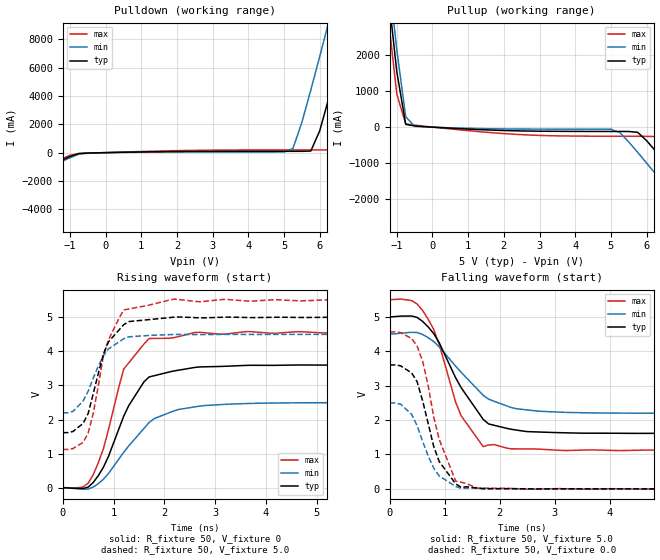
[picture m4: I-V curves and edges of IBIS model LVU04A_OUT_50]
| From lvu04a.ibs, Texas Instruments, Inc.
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|   Model LVU04A_OUT_50
[Model]   LVU04A_OUT_50
Model_type  Output
Polarity   Inverting
Vmeas = 2.50v
Cref = 15pf
| variable   typ   min   max
C_comp   6.50pf   4.88pf   8.13pf
[Temperature Range]   25   85   -40
[Voltage Range]   5.0   4.5   5.5
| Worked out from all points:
|   slope of the pulldown table from 0 to 0.75 V, typ, clamps not added: 19.9 ohm
|   slope of the pullup table from 0 to 0.75 V, typ, clamps not added: 17.9 ohm
|   rising waveform, R_fixture 50, V_fixture 0: 20-80 % time 664ps typ, 834ps min, 547ps max; typ from 0 V to 3.6 V
|   falling waveform, R_fixture 50, V_fixture 5.0: 20-80 % time 709ps typ, 805ps min, 553ps max; typ from 5 V to 1.61 V
|   rising waveform, R_fixture 50, V_fixture 5.0: 20-80 % time 405ps typ, 443ps min, 425ps max; typ from 1.61 V to 5 V
|   falling waveform, R_fixture 50, V_fixture 0.0: 20-80 % time 394ps typ, 395ps min, 422ps max; typ from 3.6 V to 0 V
[Pulldown]
|   Voltage   I(typ)   I(min)   I(max)
-5V       -5.137A    -5.221A    -5.049A
-750mV    -58.91mA   -107.9mA   -71.34mA
5V        93.29mA    48.15mA    192mA
5.25V     93.34mA    298.4mA    192.2mA
5.75V     115.9mA    4.416A     192.3mA
6V        1.543A     6.782A     192.5mA
6.25V     3.802A     9.188A     193.6mA
6.5V      6.175A     11.62A     931.3mA
6.75V     8.589A     14.06A     3.152A
7.25V     13.47A     18.96A     7.958A
7.5V      15.93A     21.43A     10.4A
10V       40.69A     46.19A     35.16A
[Pullup]
|   Voltage   I(typ)   I(min)   I(max)
-5V       40.69A     41.22A     40.13A
-1.25V    3.8A       4.415A     3.147A
-1V       1.538A     2.141A     913.8mA
-750mV    77.31mA    289.2mA    88.2mA
-500mV    33.52mA    21.54mA    56.26mA
5V        -119.7mA   -57.82mA   -252.2mA
5.75V     -143.8mA   -698.4mA   -252.6mA
6.25V     -660.6mA   -1.294A    -261mA
7.5V      -2.169A    -2.814A    -1.581A
8V        -2.781A    -3.427A    -2.192A
8.5V      -3.395A    -4.041A    -2.806A
10V       -5.243A    -5.888A    -4.654A
[Ramp]
| variable   typ   min   max
dV/dt_r  2.1615E+00/6.4572E-10  1.4987E+00/8.5844E-10  2.7383E+00/5.0255E-10
dV/dt_f  2.0525E+00/6.3930E-10  1.4118E+00/8.3550E-10  2.6399E+00/5.4668E-10
R_load = 50
[Rising Waveform]
R_fixture = 50
V_fixture = 0
|   Time   V(typ)   V(min)   V(max)
0s        0V         0V         0V
400ps     -27.85mV   -45.29mV   16mV
600ps     151.8mV    16.63mV    380.7mV
800ps     599mV      246.5mV    1.142V
1.2ns     2.099V     1.038V     3.482V
1.6ns     3.11V      1.741V     4.22V
1.8ns     3.287V     2.027V     4.381V
2.6ns     3.53V      2.372V     4.554V
4.8ns     3.601V     2.492V     4.57V
25ns      3.602V     2.498V     4.561V
[Falling Waveform]
R_fixture = 50
V_fixture = 5.0
V_fixture_min = 4.5
V_fixture_max = 5.5
|   Time   V(typ)   V(min)   V(max)
0s        5V         4.5V       5.5V
400ps     5.026V     4.552V     5.475V
600ps     4.869V     4.489V     5.184V
900ps     4.252V     4.132V     4.209V
1.2ns     3.228V     3.567V     2.518V
1.3ns     2.942V     3.389V     2.124V
1.7ns     2.021V     2.72V      1.229V
2.3ns     1.711V     2.331V     1.163V
3.7ns     1.619V     2.208V     1.133V
25ns      1.614V     2.199V     1.122V
[Rising Waveform]
R_fixture = 50
V_fixture = 5.0
V_fixture_min = 4.5
V_fixture_max = 5.5
|   Time   V(typ)   V(min)   V(max)
0s        1.614V     2.199V     1.122V
200ps     1.648V     2.237V     1.146V
400ps     1.885V     2.544V     1.329V
500ps     2.176V     2.83V      1.599V
600ps     2.76V      3.219V     2.183V
800ps     3.917V     3.873V     3.897V
900ps     4.281V     4.074V     4.339V
1.2ns     4.785V     4.374V     5.22V
2.2ns     5.007V     4.497V     5.538V
25ns      5V         4.5V       5.5V
[Falling Waveform]
R_fixture = 50
V_fixture = 0.0
|   Time   V(typ)   V(min)   V(max)
0s        3.602V     2.498V     4.561V
200ps     3.577V     2.464V     4.543V
400ps     3.37V      2.163V     4.372V
500ps     3.113V     1.837V     4.147V
600ps     2.555V     1.375V     3.71V
800ps     1.238V     605mV      2.098V
900ps     796.7mV    375.9mV    1.442V
1.2ns     146.6mV    69.17mV    224.7mV
1.6ns     21.55mV    18.9mV     21.77mV
25ns      0V         0V         0V
